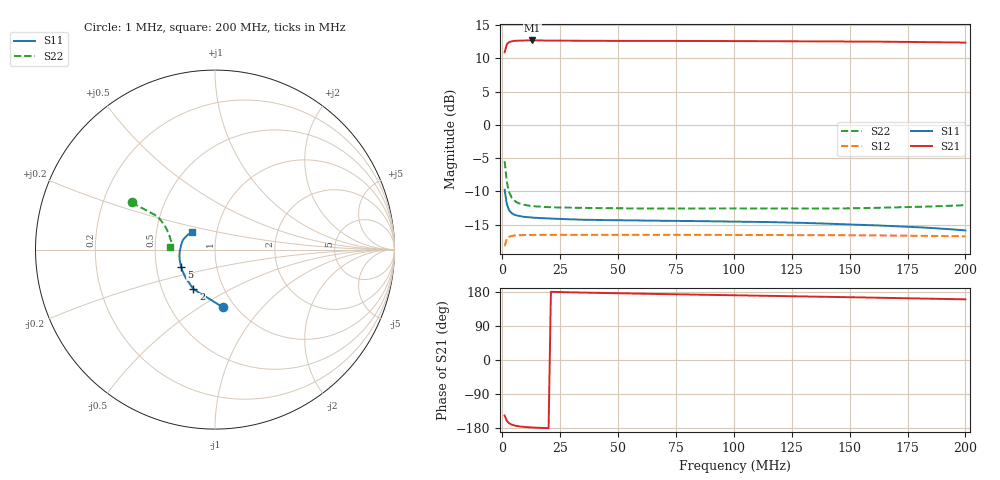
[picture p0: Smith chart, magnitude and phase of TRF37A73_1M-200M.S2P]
!Agilent Technologies,E5071B,JP1KK00322,A.09.10
!Date: Mon Jul 07 16:42:24 2014
!Data & Calibration Information:
!Freq		S11:SOLT2(ON)  S21:SOLT2(ON)  S12:SOLT2(ON)  S22:SOLT2(ON)
# Hz S dB R 50
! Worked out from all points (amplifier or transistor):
!   200 points, 1 MHz to 200 MHz, reference 50 ohm
!   highest |S21| = 12.7 dB at 13 MHz (marker M1)
!   |S21| within 3 dB of that: start of sweep to end of sweep
!   unconditionally stable (mu >= 1): start of sweep to end of sweep
!   at 34 MHz: K = 1.08, MAG = 12.9 dB, |S12| = -16.5 dB
!   at 101 MHz: K = 1.08, MAG = 12.9 dB, |S12| = -16.6 dB
!   at 200 MHz: K = 1.10, MAG = 12.7 dB, |S12| = -16.8 dB
!   S11 on the Smith chart (normalised r, x): 1 MHz: 0.88, -0.63; 2 MHz: 0.72, -0.34; 5 MHz: 0.67, -0.13; 200 MHz: 0.76, +0.15
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1000000  -9.76 -82.0  10.92 -146.6  -18.26 36.7  -5.45 150.5
2000000  -12.01 -118.6  12.17 -161.2  -17.12 20.2  -8.67 149.9
3000000  -12.88 -136.4  12.46 -167.2  -16.84 13.8  -10.17 154.5
4000000  -13.27 -146.5  12.58 -170.4  -16.73 10.5  -10.92 158.6
5000000  -13.49 -153.0  12.64 -172.4  -16.67 8.3  -11.34 161.6
6000000  -13.61 -157.6  12.67 -173.8  -16.64 6.8  -11.60 163.9
7000000  -13.70 -160.9  12.68 -174.8  -16.61 5.8  -11.78 165.6
8000000  -13.77 -163.5  12.69 -175.7  -16.60 4.9  -11.91 167.0
1e7  -13.86 -167.2  12.71 -176.9  -16.58 3.7  -12.08 169.0
1.3e7  -13.95 -170.9  12.71 -178.1  -16.56 2.5  -12.22 171.0
1.6e7  -14.02 -173.4  12.71 -179.0  -16.55 1.6  -12.31 172.2
2.2e7  -14.12 -176.7  12.70 179.7  -16.54 0.4  -12.41 173.7
2.9e7  -14.21 -179.4  12.68 178.6  -16.53 -0.6  -12.46 174.7
3.5e7  -14.27 178.8  12.66 177.8  -16.53 -1.3  -12.50 175.1
4.4e7  -14.33 176.4  12.65 176.7  -16.53 -2.4  -12.53 175.5
6.8e7  -14.43 171.5  12.64 174.1  -16.54 -4.6  -12.60 175.9
1.01e8  -14.55 165.6  12.62 170.7  -16.56 -7.5  -12.57 175.8
1.34e8  -14.80 159.7  12.58 167.4  -16.60 -10.3  -12.58 175.8
1.51e8  -15.00 156.3  12.55 165.6  -16.62 -11.7  -12.55 176.2
1.67e8  -15.20 152.7  12.52 163.8  -16.65 -13.3  -12.44 176.6
1.86e8  -15.54 147.6  12.46 161.7  -16.72 -15.1  -12.27 176.8
2e8  -15.89 143.2  12.39 160.1  -16.78 -16.5  -12.08 177.2
